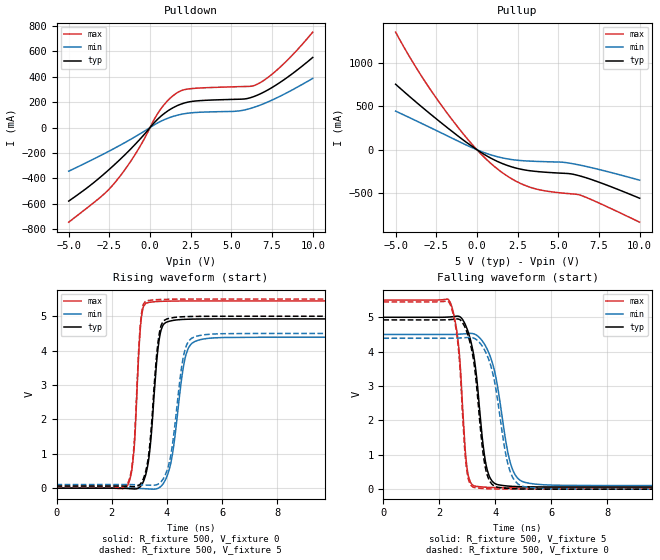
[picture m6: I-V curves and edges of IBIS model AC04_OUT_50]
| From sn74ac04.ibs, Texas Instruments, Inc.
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[Model]   AC04_OUT_50
Model_type  Output
Vref =   0
Rref =   500
Cref =   50p
Vmeas =   2.5
| variable   typ   min   max
C_comp   9.86pF   6.76pF   13.61pF
| C_pullup   10.12pF   6.76pF   13.19pF
| C_pulldown   9.61pF   6.78pF   13.61pF
[Temperature Range]   40   100   -40
| Ambient temperature   25   85   -40
[Voltage range]   5   4.5   5.5
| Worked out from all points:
|   slope of the pulldown table from 0 to 0.75 V, typ, clamps not added: 7.63 ohm
|   slope of the pullup table from 0 to 0.75 V, typ, clamps not added: 8.61 ohm
|   rising waveform, R_fixture 500, V_fixture 0: 20-80 % time 298ps typ, 418ps min, 208ps max; typ from 0 V to 4.92 V
|   falling waveform, R_fixture 500, V_fixture 5: 20-80 % time 399ps typ, 558ps min, 271ps max; typ from 5 V to 0.063 V
|   rising waveform, R_fixture 500, V_fixture 5: 20-80 % time 294ps typ, 406ps min, 209ps max; typ from 0.063 V to 5 V
|   falling waveform, R_fixture 500, V_fixture 0: 20-80 % time 391ps typ, 545ps min, 266ps max; typ from 4.92 V to 0 V
[Pulldown]
| AC04_OUT_50
|   Voltage   I(typ)   I(min)   I(max)
-5V       -580.4mA   -344.3mA   -746.8mA
-3V       -385.5mA   -218.2mA   -544mA
-2.13V    -286.2mA   -159.9mA   -429.7mA
-860mV    -125.1mA   -68.18mA   -200.6mA
550mV     75.78mA    41.96mA    126.1mA
1.45V     158.6mA    88.99mA    254.7mA
1.895V    184.2mA    103.6mA    289.5mA
2.39V     202mA      113.9mA    304.9mA
5.385V    222.9mA    129.9mA    322.1mA
6.535V    252.1mA    165.9mA    338.3mA
8.04V     360.1mA    249.9mA    481.5mA
10V       553.1mA    387.7mA    752.8mA
[Pullup]
| AC04_OUT_50
|   Voltage   I(typ)   I(min)   I(max)
-5V       757.2mA    446.5mA    1.36A
-3.49V    510.8mA    312.3mA    875.4mA
-1.795V   251.3mA    158mA      414.2mA
-115mV    14.91mA    9.349mA    23.63mA
600mV     -71.21mA   -43.73mA   -114.4mA
1.315V    -140mA     -83.59mA   -230.4mA
2.33V     -208.6mA   -118.5mA   -356.8mA
3.345V    -245mA     -132.5mA   -438.6mA
5.24V     -271.7mA   -144.4mA   -501mA
6.195V    -296.4mA   -172.6mA   -517.7mA
7.675V    -387.4mA   -236.4mA   -631mA
10V       -561.1mA   -352.2mA   -838mA
[Ramp]
| AC04_OUT_50
| variable   typ   min   max
dV/dt_r   2.97/3.11E-10   2.65/4.30E-10   3.28/2.15E-10
dV/dt_f   2.98/4.10E-10   2.66/5.71E-10   3.29/2.78E-10
R_load = 500
[Rising Waveform]
| AC04_OUT_50
R_fixture =   500
C_fixture =   0
L_fixture =   0
V_fixture =   0
V_fixture_min = 0
V_fixture_max = 0
|   Time   V(typ)   V(min)   V(max)
0s        1.299nV    2.226nV    795.1pV
2.59ns    -10.9mV    691.7uV    104.7mV
2.815ns   -23.36mV   -3.037mV   1.177V
3.075ns   83.18mV    -11.69mV   4.948V
3.36ns    954.2mV    -23.6mV    5.405V
3.845ns   4.713V     106.7mV    5.435V
4.175ns   4.871V     861.4mV    5.441V
4.705ns   4.912V     3.916V     5.445V
5.47ns    4.921V     4.355V     5.446V
50ns      4.923V     4.389V     5.446V
[Falling Waveform]
| AC04_OUT_50
R_fixture =   500
C_fixture =   0
L_fixture =   0
V_fixture =   5
V_fixture_min = 4.5
V_fixture_max = 5.5
|   Time   V(typ)   V(min)   V(max)
0s        5V         4.5V       5.5V
2.385ns   5.009V     4.499V     5.44V
2.69ns    5.029V     4.507V     4.158V
3ns       4.646V     4.526V     567.1mV
3.33ns    3.287V     4.479V     78.74mV
3.59ns    1.13V      4.249V     59.92mV
3.81ns    336.6mV    3.884V     50.68mV
4.59ns    82.43mV    636.2mV    42.36mV
5.415ns   66.35mV    148.4mV    41.08mV
50ns      63.36mV    104.1mV    40.77mV
[Rising Waveform]
| AC04_OUT_50
R_fixture =   500
C_fixture =   0
L_fixture =   0
V_fixture =   5
V_fixture_min = 4.5
V_fixture_max = 5.5
|   Time   V(typ)   V(min)   V(max)
0s        63.36mV    104.1mV    40.77mV
2.585ns   53.32mV    104.7mV    144.4mV
2.81ns    43.73mV    101.1mV    1.248V
3.07ns    154.7mV    93.72mV    5.014V
3.355ns   1.07V      86.07mV    5.462V
3.805ns   4.758V     201.3mV    5.489V
4.14ns    4.948V     946.2mV    5.495V
4.67ns    4.989V     4.062V     5.498V
5.39ns    4.998V     4.465V     5.5V
50ns      5V         4.5V       5.5V
[Falling Waveform]
| AC04_OUT_50
R_fixture =   500
C_fixture =   0
L_fixture =   0
V_fixture =   0
V_fixture_min = 0
V_fixture_max = 0
|   Time   V(typ)   V(min)   V(max)
0s        4.923V     4.389V     5.446V
2.385ns   4.932V     4.389V     5.378V
2.675ns   4.948V     4.396V     4.148V
2.975ns   4.593V     4.409V     588.1mV
3.27ns    3.475V     4.378V     41.54mV
3.56ns    1.073V     4.129V     19.32mV
3.78ns    268.2mV    3.741V     10.04mV
4.515ns   18.45mV    556.1mV    1.839mV
5.285ns   3.165mV    42.74mV    414uV
50ns      -2.587nV   -3.188nV   -5.845nV
